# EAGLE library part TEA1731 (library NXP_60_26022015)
GreenChip SMPS control IC The TEA1731LTS is a low cost Switched Mode Power Supply (SMPS) controller IC intended for flyback topologies. The TEA1731LTS operates in peak current and frequency control mode. Frequency jitter has been implemented to reduce ElectroMagnetic Interference (EMI). Slope compensation is integrated for Continuous Conduction Mode (CCM) operation. The TEA1731LTS IC features OverPower Protection (OPP). The controller accepts an overpower situation for a limited amount of time. One pin is reserved for protection purposes. OverTemperature Protection (OTP) can be implemented with a minimal number of external components. At low-power levels, the primary peak current is set to 25 % of the maximum peak current. The switching frequency is reduced to limit the switching losses. The combination of fixed frequency operation at high output power and frequency reduction at low output power provides high efficiency over the total load range. The TEA1731LTS makes the design of low cost, highly efficient and reliable supplies for power requirements up to 75 W easier by requiring a minimum number of external components. AAL Eindhoven MK
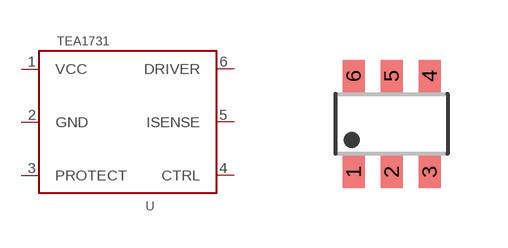
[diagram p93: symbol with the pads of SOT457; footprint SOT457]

Designator prefix U

## TEA1731LTS (12NC: 9352 965 45115), TEA1731TS (12NC: 9352 965 44115; FARNELL: 2142714)  [SOT457]
1  VCC  pwr
2  GND  in
3  PROTECT  pas
4  CTRL  in
5  ISENSE  out
6  DRIVER  pas

## Footprint SOT457 (pad centres in mm)
SOT457 TSOP6: Plastic surface-mounted package; 6 lead JEIDA: SC73 A.K.A. SOT23-6
smd 0.55 x 0.8: 1 -0.95,-1.2; 2 0,-1.2; 3 0.95,-1.2; 4 0.95,1.2; 5 0,1.2; 6 -0.95,1.2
